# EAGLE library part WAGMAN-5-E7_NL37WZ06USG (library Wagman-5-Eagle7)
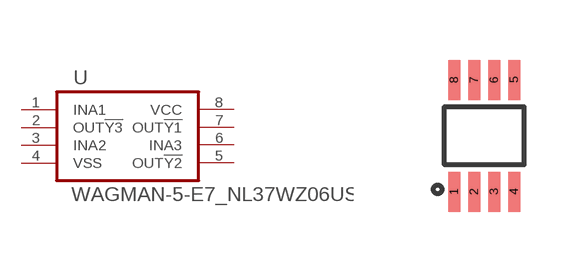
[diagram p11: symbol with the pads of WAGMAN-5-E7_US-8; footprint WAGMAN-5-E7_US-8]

Designator prefix U

## WAGMAN-5-E7_NL37WZ06USG  [WAGMAN-5-E7_US-8]
1  INA1  pwr
2  OUT!Y3  pas
3  INA2  pas
4  VSS  pas
5  OUT!Y2  pas
6  INA3  pas
7  OUT!Y1  pas
8  VCC  pas

## Footprint WAGMAN-5-E7_US-8 (pad centres in mm)
smd 0.3 x 1: 1 -0.75,-1.4; 2 -0.25,-1.4; 3 0.25,-1.4; 4 0.75,-1.4; 5 0.75,1.4; 6 0.25,1.4; 7 -0.25,1.4; 8 -0.75,1.4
